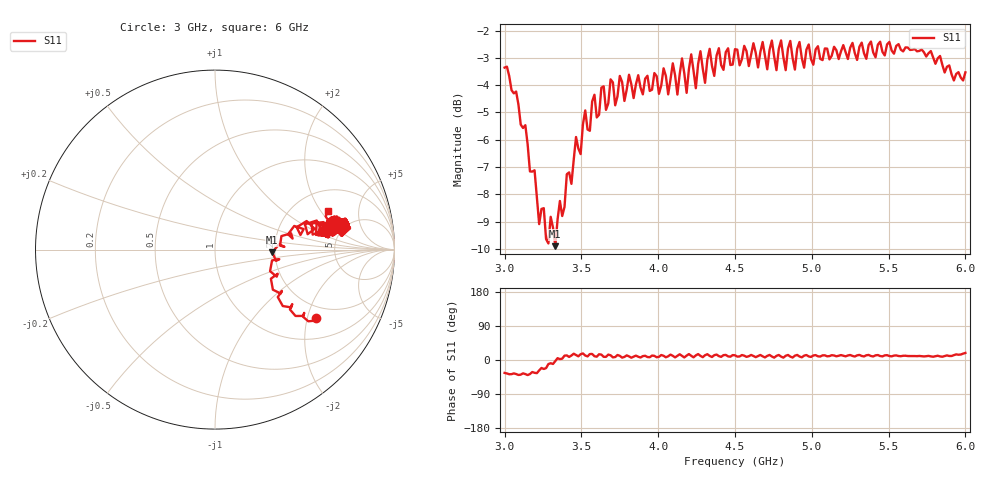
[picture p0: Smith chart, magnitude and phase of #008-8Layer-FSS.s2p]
!  05/08/2025  17:34:20
! Ref Plane: 0.000 mm
# MHZ S MA R  50
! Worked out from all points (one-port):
!   201 points, 3 GHz to 6 GHz, reference 50 ohm
!   lowest |S11| = -9.9 dB at 3.33 GHz (marker M1), VSWR 1.94, Z = 96.9 - j3.43 ohm
!   |S11| at or under -10 dB: nowhere
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3000  0.6795 -34.1
3150  0.4914 -39.8
3330  0.3199 -2.9
3375  0.3633 3.5
3510  0.5349 17.3
3750  0.656 11.0
4125  0.6064 10.9
4155  0.7063 11.0
4185  0.6108 11.6
4215  0.7185 11.1
4245  0.6229 12.2
4275  0.7281 10.9
4305  0.6372 12.7
4335  0.7354 10.8
4365  0.6561 12.7
4500  0.7345 12.4
4695  0.7148 6.8
4725  0.7324 13.3
4755  0.7122 6.2
4785  0.735 13.2
4815  0.7097 6.2
4845  0.7364 13.3
4875  0.7075 6.5
4905  0.736 13.3
4935  0.7072 7.1
5250  0.7389 13.2
5625  0.7394 10.4
6000  0.666 18.7
